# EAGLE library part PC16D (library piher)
POTENTIOMETER tandem carbon potentiometer, 16 mm, S3ROH
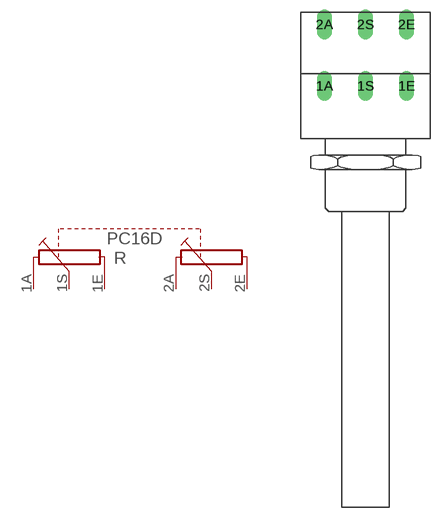
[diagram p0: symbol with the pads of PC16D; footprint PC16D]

Designator prefix R

## PC16D (OC_FARNELL: 4453049; OC_NEWARK: unknown)  [PC16D]
1A  1A  pas
1E  1E  pas
1S  1S  pas
2A  2A  pas
2E  2E  pas
2S  2S  pas

## Footprint PC16D (pad centres in mm)
POTENTIOMETER tandem carbon potentiometer, 16 mm
drill 1.2 long: 1A -5,6.5; 1E 5,6.5; 1S 0,6.5; 2A -5,14; 2E 5,14; 2S 0,14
